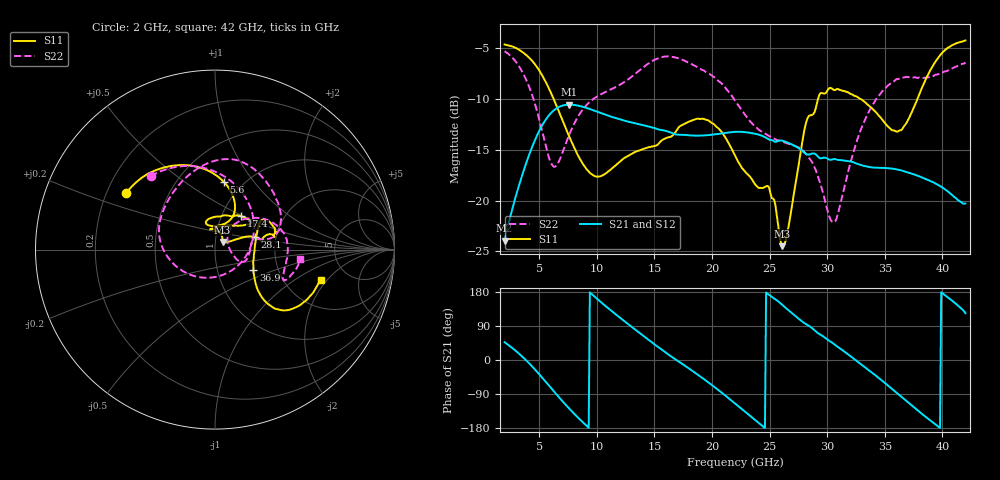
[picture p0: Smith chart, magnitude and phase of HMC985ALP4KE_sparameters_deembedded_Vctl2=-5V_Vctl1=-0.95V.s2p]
!s2p File: Measurements: S11, S21, S12, S22
# GHz S dB R 50.0
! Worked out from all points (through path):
!   401 points, 2 GHz to 42 GHz, reference 50 ohm
!   highest |S21| = -10.55 dB at 7.6 GHz (marker M1); lowest = -23.9 dB at 2 GHz (marker M2)
!   lowest |S11| = -24.5 dB at 26.1 GHz (marker M3), VSWR 1.13, Z = 54.2 + j4.59 ohm
!   |S11| at or under -10 dB: 6.26 GHz to 29.21 GHz (22.95 GHz wide, 129 % of centre); 32.91 GHz to 37.83 GHz (4.925 GHz wide, 13.9 % of centre)
!   |S22| runs from -22.1 to -5.3 dB; largest |S21 - S12| = 0.00033
!   S11 on the Smith chart (normalised r, x): 2 GHz: 0.28, +0.27; 5.6 GHz: 0.82, +0.72; 17.4 GHz: 1.23, +0.49; 28.1 GHz: 1.55, +0.23; 36.9 GHz: 1.49, -0.36; 42 GHz: 3.15, -1.74
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2  -4.62 147.6  -23.95 46.9  -23.96 46.9  -5.28 131.2
3.6  -5.42 121.0  -17.23 7.0  -17.24 7.0  -7.47 86.4
4.7  -6.68 100.1  -13.87 -27.2  -13.87 -27.2  -10.73 44.6
5.6  -8.39 82.6  -11.98 -58.6  -11.98 -58.6  -14.74 -6.3
6.4  -10.38 69.8  -11.00 -87.1  -11.01 -87.1  -16.65 -71.3
7.6  -13.67 61.8  -10.55 -127.9  -10.55 -127.9  -13.53 -143.4
8.7  -16.23 69.4  -10.73 -161.7  -10.74 -161.7  -11.16 -175.3
12  -16.17 108.9  -12.00 111.9  -12.01 111.9  -8.60 137.2
15.4  -14.36 78.6  -13.01 32.8  -13.01 32.8  -5.96 85.8
17.4  -12.56 52.1  -13.52 -9.7  -13.53 -9.7  -6.12 62.2
19.7  -12.12 36.1  -13.55 -59.4  -13.56 -59.3  -7.47 30.9
22  -15.54 53.0  -13.23 -114.8  -13.24 -114.7  -10.14 11.4
24.9  -18.60 97.8  -13.96 173.4  -13.97 173.4  -13.61 11.6
26.1  -24.49 45.0  -14.10 145.5  -14.11 145.5  -14.19 -1.5
28.1  -12.64 17.7  -15.36 95.9  -15.36 95.9  -15.34 -23.6
28.7  -11.56 10.3  -15.37 83.8  -15.37 83.8  -16.23 -25.4
30.6  -9.12 16.9  -15.91 42.0  -15.91 42.0  -22.14 20.0
33  -10.05 32.0  -16.52 -12.7  -16.53 -12.7  -12.78 46.9
35.4  -12.83 9.6  -16.82 -70.4  -16.83 -70.3  -8.56 20.3
36.9  -12.33 -27.9  -17.18 -108.7  -17.19 -108.6  -7.82 2.6
39.6  -6.01 -42.4  -18.43 -174.6  -18.43 -174.6  -7.58 -23.9
42  -4.23 -16.2  -20.29 123.5  -20.31 123.6  -6.40 -6.1
